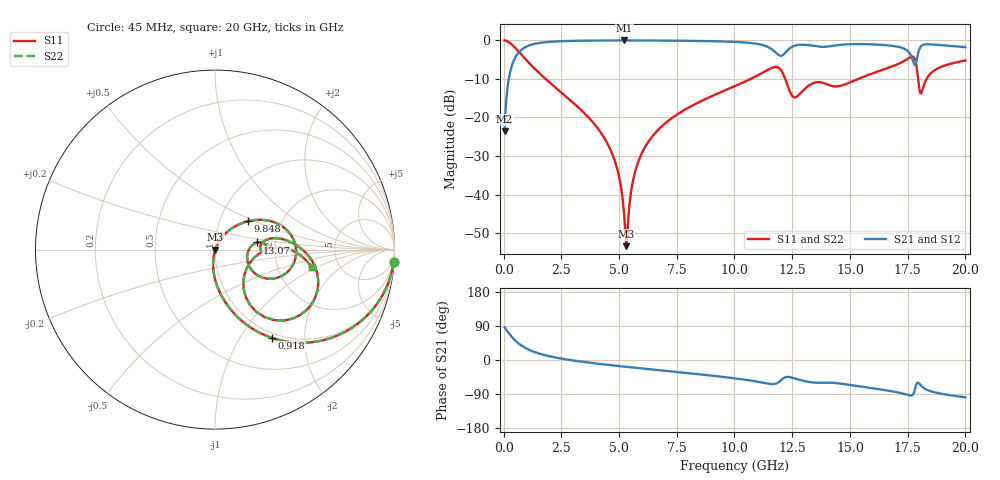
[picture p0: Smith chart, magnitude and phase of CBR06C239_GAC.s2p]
! S-parameter model data by Modelithics Inc.  support@modelithics.com 813-866-6335  Tampa FL USA
! S-Parameter data specifications:
! Substrate: 20-mil Rogers 4350B, substrate thickness, H=0.508mm, Dielectric constant, Er=3.75
! PCB Mounting Pad Footprint: Pad width, PadW=0.85mm , Pad length, PadL=0.64mm , Pad gap, PadG (edge-to-edge)=0.62mm , Reference planes=1.9mm apart
#  GHz  S  MA  R 50
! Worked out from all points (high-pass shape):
!   801 points, 45 MHz to 20 GHz, reference 50 ohm
!   highest |S21| = -0.02 dB at 5.233 GHz (marker M1); lowest = -23.6 dB at 45 MHz (marker M2)
!   |S21| within 3 dB of the highest: 671.4 MHz to 11.76 GHz (11.09 GHz wide, 178 % of centre); 12.23 GHz to 17.54 GHz (5.315 GHz wide, 35.7 % of centre)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
!   lowest |S11| = -53.4 dB at 5.308 GHz (marker M3), VSWR 1.00, Z = 50.2 - j0.113 ohm
!   |S11| at or under -10 dB: 1.822 GHz to 10.7 GHz (8.88 GHz wide, 142 % of centre); 12.2 GHz to 15.35 GHz (3.155 GHz wide, 22.9 % of centre); 17.95 GHz to 18.32 GHz (367.8 MHz wide, 2.03 % of centre)
!   |S22| runs from -53.4 to 0.0 dB; largest |S21 - S12| = 0
!   S11 on the Smith chart (normalised r, x): 45 MHz: 1, -29; 918 MHz: 0.93, -1.39; 9.848 GHz: 1.36, +0.46; 13.07 GHz: 1.61, +0.14; 20 GHz: 3.15, -0.89
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0.045  0.9978 -3.9  0.06586 86.1  0.06586 86.1  0.9978 -3.9
0.344325  0.8917 -28.1  0.452 61.9  0.452 61.9  0.8917 -28.1
0.918031  0.5852 -57.2  0.8098 32.7  0.8098 32.7  0.5852 -57.2
3.387462  0.123 -93.7  0.9905 -4.5  0.9905 -4.5  0.123 -93.7
4.734425  0.03212 -100.8  0.9973 -14.3  0.9973 -14.3  0.03212 -100.8
5.03375  0.01541 -98.7  0.9976 -16.2  0.9976 -16.2  0.01541 -98.7
5.2333  0.004939 -82.8  0.9977 -17.5  0.9977 -17.5  0.004939 -82.8
5.308131  0.002141 -31.8  0.9976 -18.0  0.9976 -18.0  0.002141 -31.8
5.782063  0.02405 63.8  0.9972 -21.0  0.9972 -21.0  0.02405 63.8
6.704981  0.06955 61.2  0.9947 -26.7  0.9947 -26.7  0.06955 61.2
9.847894  0.2425 40.7  0.9604 -47.1  0.9604 -47.1  0.2425 40.7
10.0225  0.2555 39.1  0.9556 -48.5  0.9556 -48.5  0.2555 39.1
11.79351  0.4526 -2.8  0.6911 -62.5  0.6911 -62.5  0.4526 -2.8
12.54182  0.1855 -15.0  0.838 -47.6  0.838 -47.6  0.1855 -15.0
13.06564  0.2385 9.6  0.8771 -56.1  0.8771 -56.1  0.2385 9.6
13.36496  0.2753 7.1  0.8561 -59.1  0.8561 -59.1  0.2753 7.1
16.68248  0.4426 4.1  0.8603 -81.2  0.8603 -81.2  0.4426 4.1
17.6054  0.6033 -17.6  0.6655 -93.8  0.6655 -93.8  0.6033 -17.6
17.82989  0.5511 -45.8  0.4776 -73.4  0.4776 -73.4  0.5511 -45.8
18.10428  0.2117 -17.4  0.8537 -69.0  0.8537 -69.0  0.2117 -17.4
18.65304  0.4072 0.4  0.8808 -85.1  0.8808 -85.1  0.4072 0.4
20  0.5485 -10.4  0.8174 -98.6  0.8174 -98.6  0.5485 -10.4
